| IBIS file stm32u535_545_ufqfpn48.ibs
[IBIS ver] 4.2
[File name] stm32u535_545_ufqfpn48.ibs
[File Rev] rev1.0
[Date]  11-09-2023
[Source] Data Created at STMicroelectronics
[Notes]  File originated from ELDO simulations.
[Disclaimer]  This information is for modeling purpose only and is
   not guaranteed. The information is subject to change without
   notice.
[Copyright] Copyright 2023 STMicroelectronics Inc.
|   Component stm32u535_545_ufqfpn48
[Component] stm32u535_545_ufqfpn48
[Manufacturer] STMicroelectronics
[Package]
| variable   typ   min   max
R_pkg  0  NA  NA
L_pkg  0  NA  NA
C_pkg  0  NA  NA
[Pin]   signal_name   model_name
1  VBAT  power
2  PC13  io8_100m_ft_v33
3  PC14-OSC32_IN  io8_100m_tamp_ft
4  PC15-OSC32_OUT  io8_100m_tamp_ft
5  PH0-OSC_IN  io8_100m_ft
6  PH1-OSC_OUT  io8_100m_ft
7  NRST  nc
8  VSSA  nc
9  VDDA  power
10  PA0  io8_100m_hslv_tamp_ft
11  PA1  io8_100m_hslv_tamp_ft
12  PA2  io8_100m_hslv_ft
13  PA3  io8_166m_hslv_ft
14  PA4  io8_100m_hslv_ft
15  PA5  io8_100m_ft
16  PA6  io8_100m_hslv_ft
17  PA7  io8_100m_hslv_i2c_ft
18  PB0  io8_100m_hslv_ft
19  PB1  io8_100m_hslv_ft
20  PB2  io8_100m_hslv_tamp_ft
21  PB10  io8_166m_hslv_i2c_ft
22  VCAP  nc
23  VSS  gnd
24  VDD  power
25  PB12  io8_166m_hslv_ft
26  PB13  io8_100m_i2c_ft
27  PB14  io8_100m_i2c_ft
28  PB15  io8_100m_ft
29  PA8  io8_166m_hslv_ft
30  PA9  io8_100m_ft
31  PA10  io8_100m_ft
32  PA11  io8_usb_ft
33  PA12  io8_usb_ft
34  PA13  io8_100m_ft
35  VSS  gnd
36  VDD  power
37  PA14  io8_100m_ft
38  PA15  io8_100m_ft
39  PB3  io8_100m_i2c_ft
40  PB4  io8_100m_i2c_ft
41  PB5  io8_166m_hslv_ft
42  PB6  io8_100m_i2c_ft
43  PB7  io8_166m_hslv_i2c_ft
44  PH3-BOOT0  io8_100m_ft
45  PB8  io8_100m_hslv_i2c_ft
46  PB9  io8_100m_hslv_i2c_ft
47  VSS  gnd
48  VDD  power
[Package Model]   455-qfpn-7x7-48-ldo-230504
[Pin Mapping]   pulldown_ref   pullup_ref   | Comment
1  nc  vsw
2  gndio  vddiom  | Depending on IO usage
| 2  gndio  vsw  | Depending on IO usage
3  gndio  vddiom  | Depending on IO usage
| 3  gndio  vsw  | Depending on IO usage
4  gndio  vddiom  | Depending on IO usage
| 4  gndio  vsw  | Depending on IO usage
5  gndio  vddiom
6  gndio  vddiom
7  nc   nc
8  nc  nc
9  nc  vddiom
10  gndio  vddiom
11  gndio  vddiom
12  gndio  vddiom
13  gndio  vddiom
14  gndio  vddiom
15  gndio  vddiom
16  gndio  vddiom
17  gndio  vddiom
18  gndio  vddiom
19  gndio  vddiom
20  gndio  vddiom
21  gndio  vddiom
22  nc  nc
23  gndio  nc
24  nc  vddiom
25  gndio  vddiom
26  gndio  vddiom
27  gndio  vddiom
28  gndio  vddiom
29  gndio  vddiom
30  gndio  vddiom  | Depending on IO usage
| 30  gndio  vddusb  | Depending on IO usage
31  gndio  vddiom  | Depending on IO usage
| 31  gndio  vddusb  | Depending on IO usage
32  gndio  vddiom  | Depending on IO usage
| 32  gndio  vddusb  | Depending on IO usage
33  gndio  vddiom  | Depending on IO usage
| 33  gndio  vddusb  | Depending on IO usage
34  gndio  vddiom  | Depending on IO usage
| 34  gndio  vddusb  | Depending on IO usage
35  gndio  nc
36  nc  vddiom
37  gndio  vddiom
38  gndio  vddiom
39  gndio  vddiom
40  gndio  vddiom
41  gndio  vddiom
42  gndio  vddiom
43  gndio  vddiom
44  gndio  vddiom
45  gndio  vddiom
46  gndio  vddiom
47  gndio  nc
48  nc  vddiom
[Model Selector] io8_100m_ft
io8_100m_ft_hs_1v2  "IO8_FT 100MHz high speed @ 1.2V"
io8_100m_ft_fs_1v2  "IO8_FT 100MHz fast speed @ 1.2V"
io8_100m_ft_fs_pd_1v2  "IO8_FT 100MHz fast speed @ 1.2V pulldown"
io8_100m_ft_ms_1v2  "IO8_FT 100MHz med speed @ 1.2V"
io8_100m_ft_ms_pd_1v2  "IO8_FT 100MHz med speed @ 1.2V pulldown"
io8_100m_ft_ls_1v2  "IO8_FT 100MHz low speed @ 1.2V"
io8_100m_ft_ls_pd_1v2  "IO8_FT 100MHz low speed @ 1.2V pulldown"
io8_100m_ft_hs_1v8  "IO8_FT 100MHz high speed @ 1.8V"
io8_100m_ft_hs_pd_1v8  "IO8_FT 100MHz high speed @ 1.8V pulldown"
io8_100m_ft_fs_1v8  "IO8_FT 100MHz fast speed @ 1.8V"
io8_100m_ft_fs_pd_1v8  "IO8_FT 100MHz fast speed @ 1.8V pulldown"
io8_100m_ft_ms_1v8  "IO8_FT 100MHz med speed @ 1.8V"
io8_100m_ft_ms_pd_1v8  "IO8_FT 100MHz med speed @ 1.8V pulldown"
io8_100m_ft_ls_1v8  "IO8_FT 100MHz low speed @ 1.8V"
io8_100m_ft_ls_pd_1v8  "IO8_FT 100MHz low speed @ 1.8V pulldown"
io8_100m_ft_hs_3v3  "IO8_FT 100MHz high speed @ 3.3V"
io8_100m_ft_hs_pd_3v3  "IO8_FT 100MHz high speed @ 3.3V pulldown"
io8_100m_ft_fs_3v3  "IO8_FT 100MHz fast speed @ 3.3V"
io8_100m_ft_fs_pd_3v3  "IO8_FT 100MHz fast speed @ 3.3V pulldown"
io8_100m_ft_ms_3v3  "IO8_FT 100MHz med speed @ 3.3V"
io8_100m_ft_ms_pd_3v3  "IO8_FT 100MHz med speed @ 3.3V pulldown"
io8_100m_ft_ls_3v3  "IO8_FT 100MHz low speed @ 3.3V"
io8_100m_ft_ls_pd_3v3  "IO8_FT 100MHz low speed @ 3.3V pulldown"
[Model Selector] io8_100m_hslv_ft
io8_100m_ft_hs_1v2  "IO8_FT 100MHz high speed @ 1.2V"
io8_100m_ft_hs_pu_1v2  "IO8_FT 100MHz high speed @ 1.2V pullup"
io8_100m_ft_hs_pd_1v2  "IO8_FT 100MHz high speed @ 1.2V pulldown"
io8_100m_ft_fs_1v2  "IO8_FT 100MHz fast speed @ 1.2V"
io8_100m_ft_fs_pu_1v2  "IO8_FT 100MHz fast speed @ 1.2V pullup"
io8_100m_ft_fs_pd_1v2  "IO8_FT 100MHz fast speed @ 1.2V pulldown"
io8_100m_ft_ms_1v2  "IO8_FT 100MHz med speed @ 1.2V"
io8_100m_ft_ms_pu_1v2  "IO8_FT 100MHz med speed @ 1.2V pullup"
io8_100m_ft_ms_pd_1v2  "IO8_FT 100MHz med speed @ 1.2V pulldown"
io8_100m_ft_ls_1v2  "IO8_FT 100MHz low speed @ 1.2V"
io8_100m_ft_ls_pu_1v2  "IO8_FT 100MHz low speed @ 1.2V pullup"
io8_100m_ft_ls_pd_1v2  "IO8_FT 100MHz low speed @ 1.2V pulldown"
io8_100m_ft_hs_1v8  "IO8_FT 100MHz high speed @ 1.8V"
io8_100m_ft_hs_pu_1v8  "IO8_FT 100MHz high speed @ 1.8V pullup"
io8_100m_ft_hs_pd_1v8  "IO8_FT 100MHz high speed @ 1.8V pulldown"
io8_100m_ft_fs_1v8  "IO8_FT 100MHz fast speed @ 1.8V"
io8_100m_ft_fs_pu_1v8  "IO8_FT 100MHz fast speed @ 1.8V pullup"
io8_100m_ft_fs_pd_1v8  "IO8_FT 100MHz fast speed @ 1.8V pulldown"
io8_100m_ft_ms_1v8  "IO8_FT 100MHz med speed @ 1.8V"
io8_100m_ft_ms_pu_1v8  "IO8_FT 100MHz med speed @ 1.8V pullup"
io8_100m_ft_ms_pd_1v8  "IO8_FT 100MHz med speed @ 1.8V pulldown"
io8_100m_ft_ls_1v8  "IO8_FT 100MHz low speed @ 1.8V"
io8_100m_ft_ls_pu_1v8  "IO8_FT 100MHz low speed @ 1.8V pullup"
io8_100m_ft_ls_pd_1v8  "IO8_FT 100MHz low speed @ 1.8V pulldown"
io8_100m_ft_hs_3v3  "IO8_FT 100MHz high speed @ 3.3V"
io8_100m_ft_hs_pu_3v3  "IO8_FT 100MHz high speed @ 3.3V pullup"
io8_100m_ft_hs_pd_3v3  "IO8_FT 100MHz high speed @ 3.3V pulldown"
io8_100m_ft_fs_3v3  "IO8_FT 100MHz fast speed @ 3.3V"
io8_100m_ft_fs_pu_3v3  "IO8_FT 100MHz fast speed @ 3.3V pullup"
io8_100m_ft_fs_pd_3v3  "IO8_FT 100MHz fast speed @ 3.3V pulldown"
io8_100m_ft_ms_3v3  "IO8_FT 100MHz med speed @ 3.3V"
io8_100m_ft_ms_pu_3v3  "IO8_FT 100MHz med speed @ 3.3V pullup"
io8_100m_ft_ms_pd_3v3  "IO8_FT 100MHz med speed @ 3.3V pulldown"
io8_100m_ft_ls_3v3  "IO8_FT 100MHz low speed @ 3.3V"
io8_100m_ft_ls_pu_3v3  "IO8_FT 100MHz low speed @ 3.3V pullup"
io8_100m_ft_ls_pd_3v3  "IO8_FT 100MHz low speed @ 3.3V pulldown"
io8_100m_hslv_ft_hs_1v2  "IO8_FT 100MHz HSLV high speed @ 1.2V"
io8_100m_hslv_ft_hs_pu_1v2  "IO8_FT 100MHz HSLV high speed @ 1.2V pullup"
io8_100m_hslv_ft_hs_pd_1v2  "IO8_FT 100MHz HSLV high speed @ 1.2V pulldown"
io8_100m_hslv_ft_fs_1v2  "IO8_FT 100MHz HSLV fast speed @ 1.2V"
io8_100m_hslv_ft_fs_pu_1v2  "IO8_FT 100MHz HSLV fast speed @ 1.2V pullup"
io8_100m_hslv_ft_fs_pd_1v2  "IO8_FT 100MHz HSLV fast speed @ 1.2V pulldown"
io8_100m_hslv_ft_ms_1v2  "IO8_FT 100MHz HSLV med speed @ 1.2V"
io8_100m_hslv_ft_ms_pu_1v2  "IO8_FT 100MHz HSLV med speed @ 1.2V pullup"
io8_100m_hslv_ft_ms_pd_1v2  "IO8_FT 100MHz HSLV med speed @ 1.2V pulldown"
io8_100m_hslv_ft_ls_1v2  "IO8_FT 100MHz HSLV low speed @ 1.2V"
io8_100m_hslv_ft_ls_pu_1v2  "IO8_FT 100MHz HSLV low speed @ 1.2V pullup"
io8_100m_hslv_ft_ls_pd_1v2  "IO8_FT 100MHz HSLV low speed @ 1.2V pulldown"
io8_100m_hslv_ft_hs_1v8  "IO8_FT 100MHz HSLV high speed @ 1.8V"
io8_100m_hslv_ft_hs_pu_1v8  "IO8_FT 100MHz HSLV high speed @ 1.8V pullup"
io8_100m_hslv_ft_hs_pd_1v8  "IO8_FT 100MHz HSLV high speed @ 1.8V pulldown"
io8_100m_hslv_ft_fs_1v8  "IO8_FT 100MHz HSLV fast speed @ 1.8V"
io8_100m_hslv_ft_fs_pu_1v8  "IO8_FT 100MHz HSLV fast speed @ 1.8V pullup"
io8_100m_hslv_ft_fs_pd_1v8  "IO8_FT 100MHz HSLV fast speed @ 1.8V pulldown"
io8_100m_hslv_ft_ms_1v8  "IO8_FT 100MHz HSLV med speed @ 1.8V"
io8_100m_hslv_ft_ms_pu_1v8  "IO8_FT 100MHz HSLV med speed @ 1.8V pullup"
io8_100m_hslv_ft_ms_pd_1v8  "IO8_FT 100MHz HSLV med speed @ 1.8V pulldown"
io8_100m_hslv_ft_ls_1v8  "IO8_FT 100MHz HSLV low speed @ 1.8V"
io8_100m_hslv_ft_ls_pu_1v8  "IO8_FT 100MHz HSLV low speed @ 1.8V pullup"
io8_100m_hslv_ft_ls_pd_1v8  "IO8_FT 100MHz HSLV low speed @ 1.8V pulldown"
io8_100m_hslv_ft_hs_2v5  "IO8_FT 100MHz HSLV high speed @ 2.5V"
io8_100m_hslv_ft_hs_pu_2v5  "IO8_FT 100MHz HSLV high speed @ 2.5V pullup"
io8_100m_hslv_ft_hs_pd_2v5  "IO8_FT 100MHz HSLV high speed @ 2.5V pulldown"
io8_100m_hslv_ft_fs_2v5  "IO8_FT 100MHz HSLV fast speed @ 2.5V"
io8_100m_hslv_ft_fs_pu_2v5  "IO8_FT 100MHz HSLV fast speed @ 2.5V pullup"
io8_100m_hslv_ft_fs_pd_2v5  "IO8_FT 100MHz HSLV fast speed @ 2.5V pulldown"
io8_100m_hslv_ft_ms_2v5  "IO8_FT 100MHz HSLV med speed @ 2.5V"
io8_100m_hslv_ft_ms_pu_2v5  "IO8_FT 100MHz HSLV med speed @ 2.5V pullup"
io8_100m_hslv_ft_ms_pd_2v5  "IO8_FT 100MHz HSLV med speed @ 2.5V pulldown"
io8_100m_hslv_ft_ls_2v5  "IO8_FT 100MHz HSLV low speed @ 2.5V"
io8_100m_hslv_ft_ls_pu_2v5  "IO8_FT 100MHz HSLV low speed @ 2.5V pullup"
io8_100m_hslv_ft_ls_pd_2v5  "IO8_FT 100MHz HSLV low speed @ 2.5V pulldown"
[Model Selector] io8_100m_hslv_i2c_ft
io8_100m_ft_hs_1v2  "IO8_FT 100MHz high speed @ 1.2V"
io8_100m_ft_hs_pu_1v2  "IO8_FT 100MHz high speed @ 1.2V pullup"
io8_100m_ft_hs_pd_1v2  "IO8_FT 100MHz high speed @ 1.2V pulldown"
io8_100m_ft_fs_1v2  "IO8_FT 100MHz fast speed @ 1.2V"
io8_100m_ft_fs_pu_1v2  "IO8_FT 100MHz fast speed @ 1.2V pullup"
io8_100m_ft_fs_pd_1v2  "IO8_FT 100MHz fast speed @ 1.2V pulldown"
io8_100m_ft_ms_1v2  "IO8_FT 100MHz med speed @ 1.2V"
io8_100m_ft_ms_pu_1v2  "IO8_FT 100MHz med speed @ 1.2V pullup"
io8_100m_ft_ms_pd_1v2  "IO8_FT 100MHz med speed @ 1.2V pulldown"
io8_100m_ft_ls_1v2  "IO8_FT 100MHz low speed @ 1.2V"
io8_100m_ft_ls_pu_1v2  "IO8_FT 100MHz low speed @ 1.2V pullup"
io8_100m_ft_ls_pd_1v2  "IO8_FT 100MHz low speed @ 1.2V pulldown"
io8_100m_ft_hs_1v8  "IO8_FT 100MHz high speed @ 1.8V"
io8_100m_ft_hs_pu_1v8  "IO8_FT 100MHz high speed @ 1.8V pullup"
io8_100m_ft_hs_pd_1v8  "IO8_FT 100MHz high speed @ 1.8V pulldown"
io8_100m_ft_fs_1v8  "IO8_FT 100MHz fast speed @ 1.8V"
io8_100m_ft_fs_pu_1v8  "IO8_FT 100MHz fast speed @ 1.8V pullup"
io8_100m_ft_fs_pd_1v8  "IO8_FT 100MHz fast speed @ 1.8V pulldown"
io8_100m_ft_ms_1v8  "IO8_FT 100MHz med speed @ 1.8V"
io8_100m_ft_ms_pu_1v8  "IO8_FT 100MHz med speed @ 1.8V pullup"
io8_100m_ft_ms_pd_1v8  "IO8_FT 100MHz med speed @ 1.8V pulldown"
io8_100m_ft_ls_1v8  "IO8_FT 100MHz low speed @ 1.8V"
io8_100m_ft_ls_pu_1v8  "IO8_FT 100MHz low speed @ 1.8V pullup"
io8_100m_ft_ls_pd_1v8  "IO8_FT 100MHz low speed @ 1.8V pulldown"
io8_100m_ft_hs_3v3  "IO8_FT 100MHz high speed @ 3.3V"
io8_100m_ft_hs_pu_3v3  "IO8_FT 100MHz high speed @ 3.3V pullup"
io8_100m_ft_hs_pd_3v3  "IO8_FT 100MHz high speed @ 3.3V pulldown"
io8_100m_ft_fs_3v3  "IO8_FT 100MHz fast speed @ 3.3V"
io8_100m_ft_fs_pu_3v3  "IO8_FT 100MHz fast speed @ 3.3V pullup"
io8_100m_ft_fs_pd_3v3  "IO8_FT 100MHz fast speed @ 3.3V pulldown"
io8_100m_ft_ms_3v3  "IO8_FT 100MHz med speed @ 3.3V"
io8_100m_ft_ms_pu_3v3  "IO8_FT 100MHz med speed @ 3.3V pullup"
io8_100m_ft_ms_pd_3v3  "IO8_FT 100MHz med speed @ 3.3V pulldown"
io8_100m_ft_ls_3v3  "IO8_FT 100MHz low speed @ 3.3V"
io8_100m_ft_ls_pu_3v3  "IO8_FT 100MHz low speed @ 3.3V pullup"
io8_100m_ft_ls_pd_3v3  "IO8_FT 100MHz low speed @ 3.3V pulldown"
io8_100m_hslv_ft_hs_1v2  "IO8_FT 100MHz HSLV high speed @ 1.2V"
io8_100m_hslv_ft_hs_pu_1v2  "IO8_FT 100MHz HSLV high speed @ 1.2V pullup"
io8_100m_hslv_ft_hs_pd_1v2  "IO8_FT 100MHz HSLV high speed @ 1.2V pulldown"
io8_100m_hslv_ft_fs_1v2  "IO8_FT 100MHz HSLV fast speed @ 1.2V"
io8_100m_hslv_ft_fs_pu_1v2  "IO8_FT 100MHz HSLV fast speed @ 1.2V pullup"
io8_100m_hslv_ft_fs_pd_1v2  "IO8_FT 100MHz HSLV fast speed @ 1.2V pulldown"
io8_100m_hslv_ft_ms_1v2  "IO8_FT 100MHz HSLV med speed @ 1.2V"
io8_100m_hslv_ft_ms_pu_1v2  "IO8_FT 100MHz HSLV med speed @ 1.2V pullup"
io8_100m_hslv_ft_ms_pd_1v2  "IO8_FT 100MHz HSLV med speed @ 1.2V pulldown"
io8_100m_hslv_ft_ls_1v2  "IO8_FT 100MHz HSLV low speed @ 1.2V"
io8_100m_hslv_ft_ls_pu_1v2  "IO8_FT 100MHz HSLV low speed @ 1.2V pullup"
io8_100m_hslv_ft_ls_pd_1v2  "IO8_FT 100MHz HSLV low speed @ 1.2V pulldown"
io8_100m_hslv_ft_hs_1v8  "IO8_FT 100MHz HSLV high speed @ 1.8V"
io8_100m_hslv_ft_hs_pu_1v8  "IO8_FT 100MHz HSLV high speed @ 1.8V pullup"
io8_100m_hslv_ft_hs_pd_1v8  "IO8_FT 100MHz HSLV high speed @ 1.8V pulldown"
io8_100m_hslv_ft_fs_1v8  "IO8_FT 100MHz HSLV fast speed @ 1.8V"
io8_100m_hslv_ft_fs_pu_1v8  "IO8_FT 100MHz HSLV fast speed @ 1.8V pullup"
io8_100m_hslv_ft_fs_pd_1v8  "IO8_FT 100MHz HSLV fast speed @ 1.8V pulldown"
io8_100m_hslv_ft_ms_1v8  "IO8_FT 100MHz HSLV med speed @ 1.8V"
io8_100m_hslv_ft_ms_pu_1v8  "IO8_FT 100MHz HSLV med speed @ 1.8V pullup"
io8_100m_hslv_ft_ms_pd_1v8  "IO8_FT 100MHz HSLV med speed @ 1.8V pulldown"
io8_100m_hslv_ft_ls_1v8  "IO8_FT 100MHz HSLV low speed @ 1.8V"
io8_100m_hslv_ft_ls_pu_1v8  "IO8_FT 100MHz HSLV low speed @ 1.8V pullup"
io8_100m_hslv_ft_ls_pd_1v8  "IO8_FT 100MHz HSLV low speed @ 1.8V pulldown"
io8_100m_hslv_ft_hs_2v5  "IO8_FT 100MHz HSLV high speed @ 2.5V"
io8_100m_hslv_ft_hs_pu_2v5  "IO8_FT 100MHz HSLV high speed @ 2.5V pullup"
io8_100m_hslv_ft_hs_pd_2v5  "IO8_FT 100MHz HSLV high speed @ 2.5V pulldown"
io8_100m_hslv_ft_fs_2v5  "IO8_FT 100MHz HSLV fast speed @ 2.5V"
io8_100m_hslv_ft_fs_pu_2v5  "IO8_FT 100MHz HSLV fast speed @ 2.5V pullup"
io8_100m_hslv_ft_fs_pd_2v5  "IO8_FT 100MHz HSLV fast speed @ 2.5V pulldown"
io8_100m_hslv_ft_ms_2v5  "IO8_FT 100MHz HSLV med speed @ 2.5V"
io8_100m_hslv_ft_ms_pu_2v5  "IO8_FT 100MHz HSLV med speed @ 2.5V pullup"
io8_100m_hslv_ft_ms_pd_2v5  "IO8_FT 100MHz HSLV med speed @ 2.5V pulldown"
io8_100m_hslv_ft_ls_2v5  "IO8_FT 100MHz HSLV low speed @ 2.5V"
io8_100m_hslv_ft_ls_pu_2v5  "IO8_FT 100MHz HSLV low speed @ 2.5V pullup"
io8_100m_hslv_ft_ls_pd_2v5  "IO8_FT 100MHz HSLV low speed @ 2.5V pulldown"
[Model Selector] io8_100m_hslv_tamp_ft
io8_100m_ft_hs_1v2  "IO8_FT 100MHz high speed @ 1.2V"
io8_100m_ft_hs_pu_1v2  "IO8_FT 100MHz high speed @ 1.2V pullup"
io8_100m_ft_hs_pd_1v2  "IO8_FT 100MHz high speed @ 1.2V pulldown"
io8_100m_ft_fs_1v2  "IO8_FT 100MHz fast speed @ 1.2V"
io8_100m_ft_fs_pu_1v2  "IO8_FT 100MHz fast speed @ 1.2V pullup"
io8_100m_ft_fs_pd_1v2  "IO8_FT 100MHz fast speed @ 1.2V pulldown"
io8_100m_ft_ms_1v2  "IO8_FT 100MHz med speed @ 1.2V"
io8_100m_ft_ms_pu_1v2  "IO8_FT 100MHz med speed @ 1.2V pullup"
io8_100m_ft_ms_pd_1v2  "IO8_FT 100MHz med speed @ 1.2V pulldown"
io8_100m_ft_ls_1v2  "IO8_FT 100MHz low speed @ 1.2V"
io8_100m_ft_ls_pu_1v2  "IO8_FT 100MHz low speed @ 1.2V pullup"
io8_100m_ft_ls_pd_1v2  "IO8_FT 100MHz low speed @ 1.2V pulldown"
io8_100m_ft_hs_1v8  "IO8_FT 100MHz high speed @ 1.8V"
io8_100m_ft_hs_pu_1v8  "IO8_FT 100MHz high speed @ 1.8V pullup"
io8_100m_ft_hs_pd_1v8  "IO8_FT 100MHz high speed @ 1.8V pulldown"
io8_100m_ft_fs_1v8  "IO8_FT 100MHz fast speed @ 1.8V"
io8_100m_ft_fs_pu_1v8  "IO8_FT 100MHz fast speed @ 1.8V pullup"
io8_100m_ft_fs_pd_1v8  "IO8_FT 100MHz fast speed @ 1.8V pulldown"
io8_100m_ft_ms_1v8  "IO8_FT 100MHz med speed @ 1.8V"
io8_100m_ft_ms_pu_1v8  "IO8_FT 100MHz med speed @ 1.8V pullup"
io8_100m_ft_ms_pd_1v8  "IO8_FT 100MHz med speed @ 1.8V pulldown"
io8_100m_ft_ls_1v8  "IO8_FT 100MHz low speed @ 1.8V"
io8_100m_ft_ls_pu_1v8  "IO8_FT 100MHz low speed @ 1.8V pullup"
io8_100m_ft_ls_pd_1v8  "IO8_FT 100MHz low speed @ 1.8V pulldown"
io8_100m_ft_hs_3v3  "IO8_FT 100MHz high speed @ 3.3V"
io8_100m_ft_hs_pu_3v3  "IO8_FT 100MHz high speed @ 3.3V pullup"
io8_100m_ft_hs_pd_3v3  "IO8_FT 100MHz high speed @ 3.3V pulldown"
io8_100m_ft_fs_3v3  "IO8_FT 100MHz fast speed @ 3.3V"
io8_100m_ft_fs_pu_3v3  "IO8_FT 100MHz fast speed @ 3.3V pullup"
io8_100m_ft_fs_pd_3v3  "IO8_FT 100MHz fast speed @ 3.3V pulldown"
io8_100m_ft_ms_3v3  "IO8_FT 100MHz med speed @ 3.3V"
io8_100m_ft_ms_pu_3v3  "IO8_FT 100MHz med speed @ 3.3V pullup"
io8_100m_ft_ms_pd_3v3  "IO8_FT 100MHz med speed @ 3.3V pulldown"
io8_100m_ft_ls_3v3  "IO8_FT 100MHz low speed @ 3.3V"
io8_100m_ft_ls_pu_3v3  "IO8_FT 100MHz low speed @ 3.3V pullup"
io8_100m_ft_ls_pd_3v3  "IO8_FT 100MHz low speed @ 3.3V pulldown"
io8_100m_hslv_ft_hs_1v2  "IO8_FT 100MHz HSLV high speed @ 1.2V"
io8_100m_hslv_ft_hs_pu_1v2  "IO8_FT 100MHz HSLV high speed @ 1.2V pullup"
io8_100m_hslv_ft_hs_pd_1v2  "IO8_FT 100MHz HSLV high speed @ 1.2V pulldown"
io8_100m_hslv_ft_fs_1v2  "IO8_FT 100MHz HSLV fast speed @ 1.2V"
io8_100m_hslv_ft_fs_pu_1v2  "IO8_FT 100MHz HSLV fast speed @ 1.2V pullup"
io8_100m_hslv_ft_fs_pd_1v2  "IO8_FT 100MHz HSLV fast speed @ 1.2V pulldown"
io8_100m_hslv_ft_ms_1v2  "IO8_FT 100MHz HSLV med speed @ 1.2V"
io8_100m_hslv_ft_ms_pu_1v2  "IO8_FT 100MHz HSLV med speed @ 1.2V pullup"
io8_100m_hslv_ft_ms_pd_1v2  "IO8_FT 100MHz HSLV med speed @ 1.2V pulldown"
io8_100m_hslv_ft_ls_1v2  "IO8_FT 100MHz HSLV low speed @ 1.2V"
io8_100m_hslv_ft_ls_pu_1v2  "IO8_FT 100MHz HSLV low speed @ 1.2V pullup"
io8_100m_hslv_ft_ls_pd_1v2  "IO8_FT 100MHz HSLV low speed @ 1.2V pulldown"
io8_100m_hslv_ft_hs_1v8  "IO8_FT 100MHz HSLV high speed @ 1.8V"
io8_100m_hslv_ft_hs_pu_1v8  "IO8_FT 100MHz HSLV high speed @ 1.8V pullup"
io8_100m_hslv_ft_hs_pd_1v8  "IO8_FT 100MHz HSLV high speed @ 1.8V pulldown"
io8_100m_hslv_ft_fs_1v8  "IO8_FT 100MHz HSLV fast speed @ 1.8V"
io8_100m_hslv_ft_fs_pu_1v8  "IO8_FT 100MHz HSLV fast speed @ 1.8V pullup"
io8_100m_hslv_ft_fs_pd_1v8  "IO8_FT 100MHz HSLV fast speed @ 1.8V pulldown"
io8_100m_hslv_ft_ms_1v8  "IO8_FT 100MHz HSLV med speed @ 1.8V"
io8_100m_hslv_ft_ms_pu_1v8  "IO8_FT 100MHz HSLV med speed @ 1.8V pullup"
io8_100m_hslv_ft_ms_pd_1v8  "IO8_FT 100MHz HSLV med speed @ 1.8V pulldown"
io8_100m_hslv_ft_ls_1v8  "IO8_FT 100MHz HSLV low speed @ 1.8V"
io8_100m_hslv_ft_ls_pu_1v8  "IO8_FT 100MHz HSLV low speed @ 1.8V pullup"
io8_100m_hslv_ft_ls_pd_1v8  "IO8_FT 100MHz HSLV low speed @ 1.8V pulldown"
io8_100m_hslv_ft_hs_2v5  "IO8_FT 100MHz HSLV high speed @ 2.5V"
io8_100m_hslv_ft_hs_pu_2v5  "IO8_FT 100MHz HSLV high speed @ 2.5V pullup"
io8_100m_hslv_ft_hs_pd_2v5  "IO8_FT 100MHz HSLV high speed @ 2.5V pulldown"
io8_100m_hslv_ft_fs_2v5  "IO8_FT 100MHz HSLV fast speed @ 2.5V"
io8_100m_hslv_ft_fs_pu_2v5  "IO8_FT 100MHz HSLV fast speed @ 2.5V pullup"
io8_100m_hslv_ft_fs_pd_2v5  "IO8_FT 100MHz HSLV fast speed @ 2.5V pulldown"
io8_100m_hslv_ft_ms_2v5  "IO8_FT 100MHz HSLV med speed @ 2.5V"
io8_100m_hslv_ft_ms_pu_2v5  "IO8_FT 100MHz HSLV med speed @ 2.5V pullup"
io8_100m_hslv_ft_ms_pd_2v5  "IO8_FT 100MHz HSLV med speed @ 2.5V pulldown"
io8_100m_hslv_ft_ls_2v5  "IO8_FT 100MHz HSLV low speed @ 2.5V"
io8_100m_hslv_ft_ls_pu_2v5  "IO8_FT 100MHz HSLV low speed @ 2.5V pullup"
io8_100m_hslv_ft_ls_pd_2v5  "IO8_FT 100MHz HSLV low speed @ 2.5V pulldown"
io8_ft_v33_hs_1v2  "IO8_FT_V33 high speed @ 1.2V"
io8_ft_v33_hs_pu_1v2  "IO8_FT_V33 high speed @ 1.2V pullup"
io8_ft_v33_hs_pd_1v2  "IO8_FT_V33 high speed @ 1.2V pulldown"
io8_ft_v33_fs_1v2  "IO8_FT_V33 fast speed @ 1.2V"
io8_ft_v33_fs_pu_1v2  "IO8_FT_V33 fast speed @ 1.2V pullup"
io8_ft_v33_fs_pd_1v2  "IO8_FT_V33 fast speed @ 1.2V pulldown"
io8_ft_v33_ms_1v2  "IO8_FT_V33 med speed @ 1.2V"
io8_ft_v33_ms_pu_1v2  "IO8_FT_V33 med speed @ 1.2V pullup"
io8_ft_v33_ms_pd_1v2  "IO8_FT_V33 med speed @ 1.2V pulldown"
io8_ft_v33_ls_1v2  "IO8_FT_V33 low speed @ 1.2V"
io8_ft_v33_ls_pu_1v2  "IO8_FT_V33 low speed @ 1.2V pullup"
io8_ft_v33_ls_pd_1v2  "IO8_FT_V33 low speed @ 1.2V pulldown"
io8_ft_v33_hs_1v8  "IO8_FT_V33 high speed @ 1.8V"
io8_ft_v33_hs_pu_1v8  "IO8_FT_V33 high speed @ 1.8V pullup"
io8_ft_v33_hs_pd_1v8  "IO8_FT_V33 high speed @ 1.8V pulldown"
io8_ft_v33_fs_1v8  "IO8_FT_V33 fast speed @ 1.8V"
io8_ft_v33_fs_pu_1v8  "IO8_FT_V33 fast speed @ 1.8V pullup"
io8_ft_v33_fs_pd_1v8  "IO8_FT_V33 fast speed @ 1.8V pulldown"
io8_ft_v33_ms_1v8  "IO8_FT_V33 med speed @ 1.8V"
io8_ft_v33_ms_pu_1v8  "IO8_FT_V33 med speed @ 1.8V pullup"
io8_ft_v33_ms_pd_1v8  "IO8_FT_V33 med speed @ 1.8V pulldown"
io8_ft_v33_ls_1v8  "IO8_FT_V33 low speed @ 1.8V"
io8_ft_v33_ls_pu_1v8  "IO8_FT_V33 low speed @ 1.8V pullup"
io8_ft_v33_ls_pd_1v8  "IO8_FT_V33 low speed @ 1.8V pulldown"
io8_ft_v33_hs_3v3  "IO8_FT_V33 high speed @ 3.3V"
io8_ft_v33_hs_pu_3v3  "IO8_FT_V33 high speed @ 3.3V pullup"
io8_ft_v33_hs_pd_3v3  "IO8_FT_V33 high speed @ 3.3V pulldown"
io8_ft_v33_fs_3v3  "IO8_FT_V33 fast speed @ 3.3V"
io8_ft_v33_fs_pu_3v3  "IO8_FT_V33 fast speed @ 3.3V pullup"
io8_ft_v33_fs_pd_3v3  "IO8_FT_V33 fast speed @ 3.3V pulldown"
io8_ft_v33_ms_3v3  "IO8_FT_V33 med speed @ 3.3V"
io8_ft_v33_ms_pu_3v3  "IO8_FT_V33 med speed @ 3.3V pullup"
io8_ft_v33_ms_pd_3v3  "IO8_FT_V33 med speed @ 3.3V pulldown"
io8_ft_v33_ls_3v3  "IO8_FT_V33 low speed @ 3.3V"
io8_ft_v33_ls_pu_3v3  "IO8_FT_V33 low speed @ 3.3V pullup"
io8_ft_v33_ls_pd_3v3  "IO8_FT_V33 low speed @ 3.3V pulldown"
[Model Selector] io8_100m_i2c_ft
io8_100m_ft_hs_1v2  "IO8_FT 100MHz high speed @ 1.2V"
io8_100m_ft_hs_pu_1v2  "IO8_FT 100MHz high speed @ 1.2V pullup"
io8_100m_ft_hs_pd_1v2  "IO8_FT 100MHz high speed @ 1.2V pulldown"
io8_100m_ft_fs_1v2  "IO8_FT 100MHz fast speed @ 1.2V"
io8_100m_ft_fs_pu_1v2  "IO8_FT 100MHz fast speed @ 1.2V pullup"
io8_100m_ft_fs_pd_1v2  "IO8_FT 100MHz fast speed @ 1.2V pulldown"
io8_100m_ft_ms_1v2  "IO8_FT 100MHz med speed @ 1.2V"
io8_100m_ft_ms_pu_1v2  "IO8_FT 100MHz med speed @ 1.2V pullup"
io8_100m_ft_ms_pd_1v2  "IO8_FT 100MHz med speed @ 1.2V pulldown"
io8_100m_ft_ls_1v2  "IO8_FT 100MHz low speed @ 1.2V"
io8_100m_ft_ls_pu_1v2  "IO8_FT 100MHz low speed @ 1.2V pullup"
io8_100m_ft_ls_pd_1v2  "IO8_FT 100MHz low speed @ 1.2V pulldown"
io8_100m_ft_hs_1v8  "IO8_FT 100MHz high speed @ 1.8V"
io8_100m_ft_hs_pu_1v8  "IO8_FT 100MHz high speed @ 1.8V pullup"
io8_100m_ft_hs_pd_1v8  "IO8_FT 100MHz high speed @ 1.8V pulldown"
io8_100m_ft_fs_1v8  "IO8_FT 100MHz fast speed @ 1.8V"
io8_100m_ft_fs_pu_1v8  "IO8_FT 100MHz fast speed @ 1.8V pullup"
io8_100m_ft_fs_pd_1v8  "IO8_FT 100MHz fast speed @ 1.8V pulldown"
io8_100m_ft_ms_1v8  "IO8_FT 100MHz med speed @ 1.8V"
io8_100m_ft_ms_pu_1v8  "IO8_FT 100MHz med speed @ 1.8V pullup"
io8_100m_ft_ms_pd_1v8  "IO8_FT 100MHz med speed @ 1.8V pulldown"
io8_100m_ft_ls_1v8  "IO8_FT 100MHz low speed @ 1.8V"
io8_100m_ft_ls_pu_1v8  "IO8_FT 100MHz low speed @ 1.8V pullup"
io8_100m_ft_ls_pd_1v8  "IO8_FT 100MHz low speed @ 1.8V pulldown"
io8_100m_ft_hs_3v3  "IO8_FT 100MHz high speed @ 3.3V"
io8_100m_ft_hs_pu_3v3  "IO8_FT 100MHz high speed @ 3.3V pullup"
io8_100m_ft_hs_pd_3v3  "IO8_FT 100MHz high speed @ 3.3V pulldown"
io8_100m_ft_fs_3v3  "IO8_FT 100MHz fast speed @ 3.3V"
io8_100m_ft_fs_pu_3v3  "IO8_FT 100MHz fast speed @ 3.3V pullup"
io8_100m_ft_fs_pd_3v3  "IO8_FT 100MHz fast speed @ 3.3V pulldown"
io8_100m_ft_ms_3v3  "IO8_FT 100MHz med speed @ 3.3V"
io8_100m_ft_ms_pu_3v3  "IO8_FT 100MHz med speed @ 3.3V pullup"
io8_100m_ft_ms_pd_3v3  "IO8_FT 100MHz med speed @ 3.3V pulldown"
io8_100m_ft_ls_3v3  "IO8_FT 100MHz low speed @ 3.3V"
io8_100m_ft_ls_pu_3v3  "IO8_FT 100MHz low speed @ 3.3V pullup"
io8_100m_ft_ls_pd_3v3  "IO8_FT 100MHz low speed @ 3.3V pulldown"
io8_100m_i2c_ft_1v2  "IO8_FT 100MHz I2C @ 1.2V"
io8_100m_i2c_ft_pu_1v2  "IO8_FT 100MHz I2C @ 1.2V pullup"
io8_100m_i2c_ft_pd_1v2  "IO8_FT 100MHz I2C @ 1.2V pulldown"
io8_100m_i2c_ft_1v8  "IO8_FT 100MHz I2C @ 1.8V"
io8_100m_i2c_ft_pu_1v8  "IO8_FT 100MHz I2C @ 1.8V pullup"
io8_100m_i2c_ft_pd_1v8  "IO8_FT 100MHz I2C @ 1,8V pulldown"
io8_100m_i2c_ft_3v3  "IO8_FT 100MHz I2C @ 3.3V"
io8_100m_i2c_ft_pu_3v3  "IO8_FT 100MHz I2C HSLV @ 3.3V pullup"
io8_100m_i2c_ft_pd_3v3  "IO8_FT 100MHz I2C @ 3.3V pulldown"
[Model Selector] io8_100m_tamp_ft
io8_100m_ft_hs_1v2  "IO8_FT 100MHz high speed @ 1.2V"
io8_100m_ft_hs_pu_1v2  "IO8_FT 100MHz high speed @ 1.2V pullup"
io8_100m_ft_hs_pd_1v2  "IO8_FT 100MHz high speed @ 1.2V pulldown"
io8_100m_ft_fs_1v2  "IO8_FT 100MHz fast speed @ 1.2V"
io8_100m_ft_fs_pu_1v2  "IO8_FT 100MHz fast speed @ 1.2V pullup"
io8_100m_ft_fs_pd_1v2  "IO8_FT 100MHz fast speed @ 1.2V pulldown"
io8_100m_ft_ms_1v2  "IO8_FT 100MHz med speed @ 1.2V"
io8_100m_ft_ms_pu_1v2  "IO8_FT 100MHz med speed @ 1.2V pullup"
io8_100m_ft_ms_pd_1v2  "IO8_FT 100MHz med speed @ 1.2V pulldown"
io8_100m_ft_ls_1v2  "IO8_FT 100MHz low speed @ 1.2V"
io8_100m_ft_ls_pu_1v2  "IO8_FT 100MHz low speed @ 1.2V pullup"
io8_100m_ft_ls_pd_1v2  "IO8_FT 100MHz low speed @ 1.2V pulldown"
io8_100m_ft_hs_1v8  "IO8_FT 100MHz high speed @ 1.8V"
io8_100m_ft_hs_pu_1v8  "IO8_FT 100MHz high speed @ 1.8V pullup"
io8_100m_ft_hs_pd_1v8  "IO8_FT 100MHz high speed @ 1.8V pulldown"
io8_100m_ft_fs_1v8  "IO8_FT 100MHz fast speed @ 1.8V"
io8_100m_ft_fs_pu_1v8  "IO8_FT 100MHz fast speed @ 1.8V pullup"
io8_100m_ft_fs_pd_1v8  "IO8_FT 100MHz fast speed @ 1.8V pulldown"
io8_100m_ft_ms_1v8  "IO8_FT 100MHz med speed @ 1.8V"
io8_100m_ft_ms_pu_1v8  "IO8_FT 100MHz med speed @ 1.8V pullup"
io8_100m_ft_ms_pd_1v8  "IO8_FT 100MHz med speed @ 1.8V pulldown"
io8_100m_ft_ls_1v8  "IO8_FT 100MHz low speed @ 1.8V"
io8_100m_ft_ls_pu_1v8  "IO8_FT 100MHz low speed @ 1.8V pullup"
io8_100m_ft_ls_pd_1v8  "IO8_FT 100MHz low speed @ 1.8V pulldown"
io8_100m_ft_hs_3v3  "IO8_FT 100MHz high speed @ 3.3V"
io8_100m_ft_hs_pu_3v3  "IO8_FT 100MHz high speed @ 3.3V pullup"
io8_100m_ft_hs_pd_3v3  "IO8_FT 100MHz high speed @ 3.3V pulldown"
io8_100m_ft_fs_3v3  "IO8_FT 100MHz fast speed @ 3.3V"
io8_100m_ft_fs_pu_3v3  "IO8_FT 100MHz fast speed @ 3.3V pullup"
io8_100m_ft_fs_pd_3v3  "IO8_FT 100MHz fast speed @ 3.3V pulldown"
io8_100m_ft_ms_3v3  "IO8_FT 100MHz med speed @ 3.3V"
io8_100m_ft_ms_pu_3v3  "IO8_FT 100MHz med speed @ 3.3V pullup"
io8_100m_ft_ms_pd_3v3  "IO8_FT 100MHz med speed @ 3.3V pulldown"
io8_100m_ft_ls_3v3  "IO8_FT 100MHz low speed @ 3.3V"
io8_100m_ft_ls_pu_3v3  "IO8_FT 100MHz low speed @ 3.3V pullup"
io8_100m_ft_ls_pd_3v3  "IO8_FT 100MHz low speed @ 3.3V pulldown"
io8_ft_v33_hs_1v2  "IO8_FT_V33 high speed @ 1.2V"
io8_ft_v33_hs_pu_1v2  "IO8_FT_V33 high speed @ 1.2V pullup"
io8_ft_v33_hs_pd_1v2  "IO8_FT_V33 high speed @ 1.2V pulldown"
io8_ft_v33_fs_1v2  "IO8_FT_V33 fast speed @ 1.2V"
io8_ft_v33_fs_pu_1v2  "IO8_FT_V33 fast speed @ 1.2V pullup"
io8_ft_v33_fs_pd_1v2  "IO8_FT_V33 fast speed @ 1.2V pulldown"
io8_ft_v33_ms_1v2  "IO8_FT_V33 med speed @ 1.2V"
io8_ft_v33_ms_pu_1v2  "IO8_FT_V33 med speed @ 1.2V pullup"
io8_ft_v33_ms_pd_1v2  "IO8_FT_V33 med speed @ 1.2V pulldown"
io8_ft_v33_ls_1v2  "IO8_FT_V33 low speed @ 1.2V"
io8_ft_v33_ls_pu_1v2  "IO8_FT_V33 low speed @ 1.2V pullup"
io8_ft_v33_ls_pd_1v2  "IO8_FT_V33 low speed @ 1.2V pulldown"
io8_ft_v33_hs_1v8  "IO8_FT_V33 high speed @ 1.8V"
io8_ft_v33_hs_pu_1v8  "IO8_FT_V33 high speed @ 1.8V pullup"
io8_ft_v33_hs_pd_1v8  "IO8_FT_V33 high speed @ 1.8V pulldown"
io8_ft_v33_fs_1v8  "IO8_FT_V33 fast speed @ 1.8V"
io8_ft_v33_fs_pu_1v8  "IO8_FT_V33 fast speed @ 1.8V pullup"
io8_ft_v33_fs_pd_1v8  "IO8_FT_V33 fast speed @ 1.8V pulldown"
io8_ft_v33_ms_1v8  "IO8_FT_V33 med speed @ 1.8V"
io8_ft_v33_ms_pu_1v8  "IO8_FT_V33 med speed @ 1.8V pullup"
io8_ft_v33_ms_pd_1v8  "IO8_FT_V33 med speed @ 1.8V pulldown"
io8_ft_v33_ls_1v8  "IO8_FT_V33 low speed @ 1.8V"
io8_ft_v33_ls_pu_1v8  "IO8_FT_V33 low speed @ 1.8V pullup"
io8_ft_v33_ls_pd_1v8  "IO8_FT_V33 low speed @ 1.8V pulldown"
io8_ft_v33_hs_3v3  "IO8_FT_V33 high speed @ 3.3V"
io8_ft_v33_hs_pu_3v3  "IO8_FT_V33 high speed @ 3.3V pullup"
io8_ft_v33_hs_pd_3v3  "IO8_FT_V33 high speed @ 3.3V pulldown"
io8_ft_v33_fs_3v3  "IO8_FT_V33 fast speed @ 3.3V"
io8_ft_v33_fs_pu_3v3  "IO8_FT_V33 fast speed @ 3.3V pullup"
io8_ft_v33_fs_pd_3v3  "IO8_FT_V33 fast speed @ 3.3V pulldown"
io8_ft_v33_ms_3v3  "IO8_FT_V33 med speed @ 3.3V"
io8_ft_v33_ms_pu_3v3  "IO8_FT_V33 med speed @ 3.3V pullup"
io8_ft_v33_ms_pd_3v3  "IO8_FT_V33 med speed @ 3.3V pulldown"
io8_ft_v33_ls_3v3  "IO8_FT_V33 low speed @ 3.3V"
io8_ft_v33_ls_pu_3v3  "IO8_FT_V33 low speed @ 3.3V pullup"
io8_ft_v33_ls_pd_3v3  "IO8_FT_V33 low speed @ 3.3V pulldown"
[Model Selector] io8_usb_ft
io8_100m_ft_hs_1v2  "IO8_FT 100MHz high speed @ 1.2V"
io8_100m_ft_hs_pu_1v2  "IO8_FT 100MHz high speed @ 1.2V pullup"
io8_100m_ft_hs_pd_1v2  "IO8_FT 100MHz high speed @ 1.2V pulldown"
io8_100m_ft_fs_1v2  "IO8_FT 100MHz fast speed @ 1.2V"
io8_100m_ft_fs_pu_1v2  "IO8_FT 100MHz fast speed @ 1.2V pullup"
io8_100m_ft_fs_pd_1v2  "IO8_FT 100MHz fast speed @ 1.2V pulldown"
io8_100m_ft_ms_1v2  "IO8_FT 100MHz med speed @ 1.2V"
io8_100m_ft_ms_pu_1v2  "IO8_FT 100MHz med speed @ 1.2V pullup"
io8_100m_ft_ms_pd_1v2  "IO8_FT 100MHz med speed @ 1.2V pulldown"
io8_100m_ft_ls_1v2  "IO8_FT 100MHz low speed @ 1.2V"
io8_100m_ft_ls_pu_1v2  "IO8_FT 100MHz low speed @ 1.2V pullup"
io8_100m_ft_ls_pd_1v2  "IO8_FT 100MHz low speed @ 1.2V pulldown"
io8_100m_ft_hs_1v8  "IO8_FT 100MHz high speed @ 1.8V"
io8_100m_ft_hs_pu_1v8  "IO8_FT 100MHz high speed @ 1.8V pullup"
io8_100m_ft_hs_pd_1v8  "IO8_FT 100MHz high speed @ 1.8V pulldown"
io8_100m_ft_fs_1v8  "IO8_FT 100MHz fast speed @ 1.8V"
io8_100m_ft_fs_pu_1v8  "IO8_FT 100MHz fast speed @ 1.8V pullup"
io8_100m_ft_fs_pd_1v8  "IO8_FT 100MHz fast speed @ 1.8V pulldown"
io8_100m_ft_ms_1v8  "IO8_FT 100MHz med speed @ 1.8V"
io8_100m_ft_ms_pu_1v8  "IO8_FT 100MHz med speed @ 1.8V pullup"
io8_100m_ft_ms_pd_1v8  "IO8_FT 100MHz med speed @ 1.8V pulldown"
io8_100m_ft_ls_1v8  "IO8_FT 100MHz low speed @ 1.8V"
io8_100m_ft_ls_pu_1v8  "IO8_FT 100MHz low speed @ 1.8V pullup"
io8_100m_ft_ls_pd_1v8  "IO8_FT 100MHz low speed @ 1.8V pulldown"
io8_100m_ft_hs_3v3  "IO8_FT 100MHz high speed @ 3.3V"
io8_100m_ft_hs_pu_3v3  "IO8_FT 100MHz high speed @ 3.3V pullup"
io8_100m_ft_hs_pd_3v3  "IO8_FT 100MHz high speed @ 3.3V pulldown"
io8_100m_ft_fs_3v3  "IO8_FT 100MHz fast speed @ 3.3V"
io8_100m_ft_fs_pu_3v3  "IO8_FT 100MHz fast speed @ 3.3V pullup"
io8_100m_ft_fs_pd_3v3  "IO8_FT 100MHz fast speed @ 3.3V pulldown"
io8_100m_ft_ms_3v3  "IO8_FT 100MHz med speed @ 3.3V"
io8_100m_ft_ms_pu_3v3  "IO8_FT 100MHz med speed @ 3.3V pullup"
io8_100m_ft_ms_pd_3v3  "IO8_FT 100MHz med speed @ 3.3V pulldown"
io8_100m_ft_ls_3v3  "IO8_FT 100MHz low speed @ 3.3V"
io8_100m_ft_ls_pu_3v3  "IO8_FT 100MHz low speed @ 3.3V pullup"
io8_100m_ft_ls_pd_3v3  "IO8_FT 100MHz low speed @ 3.3V pulldown"
io8_usb_fs_3v3  "IOUSB fast speed @ 3.3V"
io8_usb_fs_pu1_3v3  "IO8USB fast speed @ 3.3V pullup1"
io8_usb_fs_pd1_3v3  "IOUSB fast speed @ 3.3V pulldown1"
io8_usb_ls_3v3  "IOUSB low speed @ 3.3V"
io8_usb_ls_pu1_3v3  "IOUSB low speed @ 3.3V pullup1"
io8_usb_ls_pd1_3v3  "IOUSB low speed @ 3.3V pulldown1"
io8_usb_fs_pu2_3v3  "IOUSB fast speed @ 3.3V pullup2"
io8_usb_fs_pd2_3v3  "IOUSB fast speed @ 3.3V pulldown2"
io8_usb_ls_pu2_3v3  "IOUSB low speed @ 3.3V pullup2"
io8_usb_ls_pd2_3v3  "IOUSB low speed @ 3.3V pulldown2"
[Model Selector] io8_166m_hslv_ft
io8_166m_ft_hs_1v2  "IO8_FT 166MHz high speed @ 1.2V"
io8_166m_ft_hs_pu_1v2  "IO8_FT 166MHz high speed @ 1.2V pullup"
io8_166m_ft_hs_pd_1v2  "IO8_FT 166MHz high speed @ 1.2V pulldown"
io8_166m_ft_fs_1v2  "IO8_FT 166MHz fast speed @ 1.2V"
io8_166m_ft_fs_pu_1v2  "IO8_FT 166MHz fast speed @ 1.2V pullup"
io8_166m_ft_fs_pd_1v2  "IO8_FT 166MHz fast speed @ 1.2V pulldown"
io8_166m_ft_ms_1v2  "IO8_FT 166MHz med speed @ 1.2V"
io8_166m_ft_ms_pu_1v2  "IO8_FT 166MHz med speed @ 1.2V pullup"
io8_166m_ft_ms_pd_1v2  "IO8_FT 166MHz med speed @ 1.2V pulldown"
io8_166m_ft_ls_1v2  "IO8_FT 166MHz low speed @ 1.2V"
io8_166m_ft_ls_pu_1v2  "IO8_FT 166MHz low speed @ 1.2V pullup"
io8_166m_ft_ls_pd_1v2  "IO8_FT 166MHz low speed @ 1.2V pulldown"
io8_166m_ft_hs_1v8  "IO8_FT 166MHz high speed @ 1.8V"
io8_166m_ft_hs_pu_1v8  "IO8_FT 166MHz high speed @ 1.8V pullup"
io8_166m_ft_hs_pd_1v8  "IO8_FT 166MHz high speed @ 1.8V pulldown"
io8_166m_ft_fs_1v8  "IO8_FT 166MHz fast speed @ 1.8V"
io8_166m_ft_fs_pu_1v8  "IO8_FT 166MHz fast speed @ 1.8V pullup"
io8_166m_ft_fs_pd_1v8  "IO8_FT 166MHz fast speed @ 1.8V pulldown"
io8_166m_ft_ms_1v8  "IO8_FT 166MHz med speed @ 1.8V"
io8_166m_ft_ms_pu_1v8  "IO8_FT 166MHz med speed @ 1.8V pullup"
io8_166m_ft_ms_pd_1v8  "IO8_FT 166MHz med speed @ 1.8V pulldown"
io8_166m_ft_ls_1v8  "IO8_FT 166MHz low speed @ 1.8V"
io8_166m_ft_ls_pu_1v8  "IO8_FT 166MHz low speed @ 1.8V pullup"
io8_166m_ft_ls_pd_1v8  "IO8_FT 166MHz low speed @ 1.8V pulldown"
io8_166m_ft_hs_3v3  "IO8_FT 166MHz high speed @ 3.3V"
io8_166m_ft_hs_pu_3v3  "IO8_FT 166MHz high speed @ 3.3V pullup"
io8_166m_ft_hs_pd_3v3  "IO8_FT 166MHz high speed @ 3.3V pulldown"
io8_166m_ft_fs_3v3  "IO8_FT 166MHz fast speed @ 3.3V"
io8_166m_ft_fs_pu_3v3  "IO8_FT 166MHz fast speed @ 3.3V pullup"
io8_166m_ft_fs_pd_3v3  "IO8_FT 166MHz fast speed @ 3.3V pulldown"
io8_166m_ft_ms_3v3  "IO8_FT 166MHz med speed @ 3.3V"
io8_166m_ft_ms_pu_3v3  "IO8_FT 166MHz med speed @ 3.3V pullup"
io8_166m_ft_ms_pd_3v3  "IO8_FT 166MHz med speed @ 3.3V pulldown"
io8_166m_ft_ls_3v3  "IO8_FT 166MHz low speed @ 3.3V"
io8_166m_ft_ls_pu_3v3  "IO8_FT 166MHz low speed @ 3.3V pullup"
io8_166m_ft_ls_pd_3v3  "IO8_FT 166MHz low speed @ 3.3V pulldown"
io8_166m_hslv_ft_hs_1v2  "IO8_FT 166MHz HSLV high speed @ 1.2V"
io8_166m_hslv_ft_hs_pu_1v2  "IO8_FT 166MHz HSLV high speed @ 1.2V pullup"
io8_166m_hslv_ft_hs_pd_1v2  "IO8_FT 166MHz HSLV high speed @ 1.2V pulldown"
io8_166m_hslv_ft_fs_1v2  "IO8_FT 166MHz HSLV fast speed @ 1.2V"
io8_166m_hslv_ft_fs_pu_1v2  "IO8_FT 166MHz HSLV fast speed @ 1.2V pullup"
io8_166m_hslv_ft_fs_pd_1v2  "IO8_FT 166MHz HSLV fast speed @ 1.2V pulldown"
io8_166m_hslv_ft_ms_1v2  "IO8_FT 166MHz HSLV med speed @ 1.2V"
io8_166m_hslv_ft_ms_pu_1v2  "IO8_FT 166MHz HSLV med speed @ 1.2V pullup"
io8_166m_hslv_ft_ms_pd_1v2  "IO8_FT 166MHz HSLV med speed @ 1.2V pulldown"
io8_166m_hslv_ft_ls_1v2  "IO8_FT 166MHz HSLV low speed @ 1.2V"
io8_166m_hslv_ft_ls_pu_1v2  "IO8_FT 166MHz HSLV low speed @ 1.2V pullup"
io8_166m_hslv_ft_ls_pd_1v2  "IO8_FT 166MHz HSLV low speed @ 1.2V pulldown"
io8_166m_hslv_ft_hs_1v8  "IO8_FT 166MHz HSLV high speed @ 1.8V"
io8_166m_hslv_ft_hs_pu_1v8  "IO8_FT 166MHz HSLV high speed @ 1.8V pullup"
io8_166m_hslv_ft_hs_pd_1v8  "IO8_FT 166MHz HSLV high speed @ 1.8V pulldown"
io8_166m_hslv_ft_fs_1v8  "IO8_FT 166MHz HSLV fast speed @ 1.8V"
io8_166m_hslv_ft_fs_pu_1v8  "IO8_FT 166MHz HSLV fast speed @ 1.8V pullup"
io8_166m_hslv_ft_fs_pd_1v8  "IO8_FT 166MHz HSLV fast speed @ 1.8V pulldown"
io8_166m_hslv_ft_ms_1v8  "IO8_FT 166MHz HSLV med speed @ 1.8V"
io8_166m_hslv_ft_ms_pu_1v8  "IO8_FT 166MHz HSLV med speed @ 1.8V pullup"
io8_166m_hslv_ft_ms_pd_1v8  "IO8_FT 166MHz HSLV med speed @ 1.8V pulldown"
io8_166m_hslv_ft_ls_1v8  "IO8_FT 166MHz HSLV low speed @ 1.8V"
io8_166m_hslv_ft_ls_pu_1v8  "IO8_FT 166MHz HSLV low speed @ 1.8V pullup"
io8_166m_hslv_ft_ls_pd_1v8  "IO8_FT 166MHz HSLV low speed @ 1.8V pulldown"
io8_166m_hslv_ft_hs_2v5  "IO8_FT 166MHz HSLV high speed @ 2.5V"
io8_166m_hslv_ft_hs_pu_2v5  "IO8_FT 166MHz HSLV high speed @ 2.5V pullup"
io8_166m_hslv_ft_hs_pd_2v5  "IO8_FT 166MHz HSLV high speed @ 2.5V pulldown"
io8_166m_hslv_ft_fs_2v5  "IO8_FT 166MHz HSLV fast speed @ 2.5V"
io8_166m_hslv_ft_fs_pu_2v5  "IO8_FT 166MHz HSLV fast speed @ 2.5V pullup"
io8_166m_hslv_ft_fs_pd_2v5  "IO8_FT 166MHz HSLV fast speed @ 2.5V pulldown"
io8_166m_hslv_ft_ms_2v5  "IO8_FT 166MHz HSLV med speed @ 2.5V"
io8_166m_hslv_ft_ms_pu_2v5  "IO8_FT 166MHz HSLV med speed @ 2.5V pullup"
io8_166m_hslv_ft_ms_pd_2v5  "IO8_FT 166MHz HSLV med speed @ 2.5V pulldown"
io8_166m_hslv_ft_ls_2v5  "IO8_FT 166MHz HSLV low speed @ 2.5V"
io8_166m_hslv_ft_ls_pu_2v5  "IO8_FT 166MHz HSLV low speed @ 2.5V pullup"
io8_166m_hslv_ft_ls_pd_2v5  "IO8_FT 166MHz HSLV low speed @ 2.5V pulldown"
[Model Selector] io8_166m_hslv_i2c_ft
io8_166m_ft_hs_1v2  "IO8_FT 166MHz high speed @ 1.2V"
io8_166m_ft_hs_pu_1v2  "IO8_FT 166MHz high speed @ 1.2V pullup"
io8_166m_ft_hs_pd_1v2  "IO8_FT 166MHz high speed @ 1.2V pulldown"
io8_166m_ft_fs_1v2  "IO8_FT 166MHz fast speed @ 1.2V"
io8_166m_ft_fs_pu_1v2  "IO8_FT 166MHz fast speed @ 1.2V pullup"
io8_166m_ft_fs_pd_1v2  "IO8_FT 166MHz fast speed @ 1.2V pulldown"
io8_166m_ft_ms_1v2  "IO8_FT 166MHz med speed @ 1.2V"
io8_166m_ft_ms_pu_1v2  "IO8_FT 166MHz med speed @ 1.2V pullup"
io8_166m_ft_ms_pd_1v2  "IO8_FT 166MHz med speed @ 1.2V pulldown"
io8_166m_ft_ls_1v2  "IO8_FT 166MHz low speed @ 1.2V"
io8_166m_ft_ls_pu_1v2  "IO8_FT 166MHz low speed @ 1.2V pullup"
io8_166m_ft_ls_pd_1v2  "IO8_FT 166MHz low speed @ 1.2V pulldown"
io8_166m_ft_hs_1v8  "IO8_FT 166MHz high speed @ 1.8V"
io8_166m_ft_hs_pu_1v8  "IO8_FT 166MHz high speed @ 1.8V pullup"
io8_166m_ft_hs_pd_1v8  "IO8_FT 166MHz high speed @ 1.8V pulldown"
io8_166m_ft_fs_1v8  "IO8_FT 166MHz fast speed @ 1.8V"
io8_166m_ft_fs_pu_1v8  "IO8_FT 166MHz fast speed @ 1.8V pullup"
io8_166m_ft_fs_pd_1v8  "IO8_FT 166MHz fast speed @ 1.8V pulldown"
io8_166m_ft_ms_1v8  "IO8_FT 166MHz med speed @ 1.8V"
io8_166m_ft_ms_pu_1v8  "IO8_FT 166MHz med speed @ 1.8V pullup"
io8_166m_ft_ms_pd_1v8  "IO8_FT 166MHz med speed @ 1.8V pulldown"
io8_166m_ft_ls_1v8  "IO8_FT 166MHz low speed @ 1.8V"
io8_166m_ft_ls_pu_1v8  "IO8_FT 166MHz low speed @ 1.8V pullup"
io8_166m_ft_ls_pd_1v8  "IO8_FT 166MHz low speed @ 1.8V pulldown"
io8_166m_ft_hs_3v3  "IO8_FT 166MHz high speed @ 3.3V"
io8_166m_ft_hs_pu_3v3  "IO8_FT 166MHz high speed @ 3.3V pullup"
io8_166m_ft_hs_pd_3v3  "IO8_FT 166MHz high speed @ 3.3V pulldown"
io8_166m_ft_fs_3v3  "IO8_FT 166MHz fast speed @ 3.3V"
io8_166m_ft_fs_pu_3v3  "IO8_FT 166MHz fast speed @ 3.3V pullup"
io8_166m_ft_fs_pd_3v3  "IO8_FT 166MHz fast speed @ 3.3V pulldown"
io8_166m_ft_ms_3v3  "IO8_FT 166MHz med speed @ 3.3V"
io8_166m_ft_ms_pu_3v3  "IO8_FT 166MHz med speed @ 3.3V pullup"
io8_166m_ft_ms_pd_3v3  "IO8_FT 166MHz med speed @ 3.3V pulldown"
io8_166m_ft_ls_3v3  "IO8_FT 166MHz low speed @ 3.3V"
io8_166m_ft_ls_pu_3v3  "IO8_FT 166MHz low speed @ 3.3V pullup"
io8_166m_ft_ls_pd_3v3  "IO8_FT 166MHz low speed @ 3.3V pulldown"
io8_166m_hslv_ft_hs_1v2  "IO8_FT 166MHz HSLV high speed @ 1.2V"
io8_166m_hslv_ft_hs_pu_1v2  "IO8_FT 166MHz HSLV high speed @ 1.2V pullup"
io8_166m_hslv_ft_hs_pd_1v2  "IO8_FT 166MHz HSLV high speed @ 1.2V pulldown"
io8_166m_hslv_ft_fs_1v2  "IO8_FT 166MHz HSLV fast speed @ 1.2V"
io8_166m_hslv_ft_fs_pu_1v2  "IO8_FT 166MHz HSLV fast speed @ 1.2V pullup"
io8_166m_hslv_ft_fs_pd_1v2  "IO8_FT 166MHz HSLV fast speed @ 1.2V pulldown"
io8_166m_hslv_ft_ms_1v2  "IO8_FT 166MHz HSLV med speed @ 1.2V"
io8_166m_hslv_ft_ms_pu_1v2  "IO8_FT 166MHz HSLV med speed @ 1.2V pullup"
io8_166m_hslv_ft_ms_pd_1v2  "IO8_FT 166MHz HSLV med speed @ 1.2V pulldown"
io8_166m_hslv_ft_ls_1v2  "IO8_FT 166MHz HSLV low speed @ 1.2V"
io8_166m_hslv_ft_ls_pu_1v2  "IO8_FT 166MHz HSLV low speed @ 1.2V pullup"
io8_166m_hslv_ft_ls_pd_1v2  "IO8_FT 166MHz HSLV low speed @ 1.2V pulldown"
io8_166m_hslv_ft_hs_1v8  "IO8_FT 166MHz HSLV high speed @ 1.8V"
io8_166m_hslv_ft_hs_pu_1v8  "IO8_FT 166MHz HSLV high speed @ 1.8V pullup"
io8_166m_hslv_ft_hs_pd_1v8  "IO8_FT 166MHz HSLV high speed @ 1.8V pulldown"
io8_166m_hslv_ft_fs_1v8  "IO8_FT 166MHz HSLV fast speed @ 1.8V"
io8_166m_hslv_ft_fs_pu_1v8  "IO8_FT 166MHz HSLV fast speed @ 1.8V pullup"
io8_166m_hslv_ft_fs_pd_1v8  "IO8_FT 166MHz HSLV fast speed @ 1.8V pulldown"
io8_166m_hslv_ft_ms_1v8  "IO8_FT 166MHz HSLV med speed @ 1.8V"
io8_166m_hslv_ft_ms_pu_1v8  "IO8_FT 166MHz HSLV med speed @ 1.8V pullup"
io8_166m_hslv_ft_ms_pd_1v8  "IO8_FT 166MHz HSLV med speed @ 1.8V pulldown"
io8_166m_hslv_ft_ls_1v8  "IO8_FT 166MHz HSLV low speed @ 1.8V"
io8_166m_hslv_ft_ls_pu_1v8  "IO8_FT 166MHz HSLV low speed @ 1.8V pullup"
io8_166m_hslv_ft_ls_pd_1v8  "IO8_FT 166MHz HSLV low speed @ 1.8V pulldown"
io8_166m_hslv_ft_hs_2v5  "IO8_FT 166MHz HSLV high speed @ 2.5V"
io8_166m_hslv_ft_hs_pu_2v5  "IO8_FT 166MHz HSLV high speed @ 2.5V pullup"
io8_166m_hslv_ft_hs_pd_2v5  "IO8_FT 166MHz HSLV high speed @ 2.5V pulldown"
io8_166m_hslv_ft_fs_2v5  "IO8_FT 166MHz HSLV fast speed @ 2.5V"
io8_166m_hslv_ft_fs_pu_2v5  "IO8_FT 166MHz HSLV fast speed @ 2.5V pullup"
io8_166m_hslv_ft_fs_pd_2v5  "IO8_FT 166MHz HSLV fast speed @ 2.5V pulldown"
io8_166m_hslv_ft_ms_2v5  "IO8_FT 166MHz HSLV med speed @ 2.5V"
io8_166m_hslv_ft_ms_pu_2v5  "IO8_FT 166MHz HSLV med speed @ 2.5V pullup"
io8_166m_hslv_ft_ms_pd_2v5  "IO8_FT 166MHz HSLV med speed @ 2.5V pulldown"
io8_166m_hslv_ft_ls_2v5  "IO8_FT 166MHz HSLV low speed @ 2.5V"
io8_166m_hslv_ft_ls_pu_2v5  "IO8_FT 166MHz HSLV low speed @ 2.5V pullup"
io8_166m_hslv_ft_ls_pd_2v5  "IO8_FT 166MHz HSLV low speed @ 2.5V pulldown"
io8_166m_i2c_ft_1v2  "IO8_FT 166MHz I2C @ 1.2V"
io8_166m_i2c_ft_pu_1v2  "IO8_FT 166MHz I2C @ 1.2V pullup"
io8_166m_i2c_ft_pd_1v2  "IO8_FT 166MHz I2C @ 1.2V pulldown"
io8_166m_i2c_ft_1v8  "IO8_FT 166MHz I2C @ 1.8V"
io8_166m_i2c_ft_pu_1v8  "IO8_FT 166MHz I2C @ 1.8V pullup"
io8_166m_i2c_ft_pd_1v8  "IO8_FT 166MHz I2C @ 1,8V pulldown"
io8_166m_i2c_ft_3v3  "IO8_FT 166MHz I2C @ 3.3V"
io8_166m_i2c_ft_pu_3v3  "IO8_FT 166MHz I2C HSLV @ 3.3V pullup"
io8_166m_i2c_ft_pd_3v3  "IO8_FT 166MHz I2C @ 3.3V pulldown"
[Model Selector] io8_100m_ft_v33
io8_ft_v33_hs_1v2  "IO8_FT_V33 high speed @ 1.2V"
io8_ft_v33_hs_pu_1v2  "IO8_FT_V33 high speed @ 1.2V pullup"
io8_ft_v33_hs_pd_1v2  "IO8_FT_V33 high speed @ 1.2V pulldown"
io8_ft_v33_fs_1v2  "IO8_FT_V33 fast speed @ 1.2V"
io8_ft_v33_fs_pu_1v2  "IO8_FT_V33 fast speed @ 1.2V pullup"
io8_ft_v33_fs_pd_1v2  "IO8_FT_V33 fast speed @ 1.2V pulldown"
io8_ft_v33_ms_1v2  "IO8_FT_V33 med speed @ 1.2V"
io8_ft_v33_ms_pu_1v2  "IO8_FT_V33 med speed @ 1.2V pullup"
io8_ft_v33_ms_pd_1v2  "IO8_FT_V33 med speed @ 1.2V pulldown"
io8_ft_v33_ls_1v2  "IO8_FT_V33 low speed @ 1.2V"
io8_ft_v33_ls_pu_1v2  "IO8_FT_V33 low speed @ 1.2V pullup"
io8_ft_v33_ls_pd_1v2  "IO8_FT_V33 low speed @ 1.2V pulldown"
io8_ft_v33_hs_1v8  "IO8_FT_V33 high speed @ 1.8V"
io8_ft_v33_hs_pu_1v8  "IO8_FT_V33 high speed @ 1.8V pullup"
io8_ft_v33_hs_pd_1v8  "IO8_FT_V33 high speed @ 1.8V pulldown"
io8_ft_v33_fs_1v8  "IO8_FT_V33 fast speed @ 1.8V"
io8_ft_v33_fs_pu_1v8  "IO8_FT_V33 fast speed @ 1.8V pullup"
io8_ft_v33_fs_pd_1v8  "IO8_FT_V33 fast speed @ 1.8V pulldown"
io8_ft_v33_ms_1v8  "IO8_FT_V33 med speed @ 1.8V"
io8_ft_v33_ms_pu_1v8  "IO8_FT_V33 med speed @ 1.8V pullup"
io8_ft_v33_ms_pd_1v8  "IO8_FT_V33 med speed @ 1.8V pulldown"
io8_ft_v33_ls_1v8  "IO8_FT_V33 low speed @ 1.8V"
io8_ft_v33_ls_pu_1v8  "IO8_FT_V33 low speed @ 1.8V pullup"
io8_ft_v33_ls_pd_1v8  "IO8_FT_V33 low speed @ 1.8V pulldown"
io8_ft_v33_hs_3v3  "IO8_FT_V33 high speed @ 3.3V"
io8_ft_v33_hs_pu_3v3  "IO8_FT_V33 high speed @ 3.3V pullup"
io8_ft_v33_hs_pd_3v3  "IO8_FT_V33 high speed @ 3.3V pulldown"
io8_ft_v33_fs_3v3  "IO8_FT_V33 fast speed @ 3.3V"
io8_ft_v33_fs_pu_3v3  "IO8_FT_V33 fast speed @ 3.3V pullup"
io8_ft_v33_fs_pd_3v3  "IO8_FT_V33 fast speed @ 3.3V pulldown"
io8_ft_v33_ms_3v3  "IO8_FT_V33 med speed @ 3.3V"
io8_ft_v33_ms_pu_3v3  "IO8_FT_V33 med speed @ 3.3V pullup"
io8_ft_v33_ms_pd_3v3  "IO8_FT_V33 med speed @ 3.3V pulldown"
io8_ft_v33_ls_3v3  "IO8_FT_V33 low speed @ 3.3V"
io8_ft_v33_ls_pu_3v3  "IO8_FT_V33 low speed @ 3.3V pullup"
io8_ft_v33_ls_pd_3v3  "IO8_FT_V33 low speed @ 3.3V pulldown"
[Define Package Model]  455-qfpn-7x7-48-ldo-230504
[Manufacturer]  Unknown
[OEM]  Unknown
[Description]  None
[Number Of Pins]  46
[Pin Numbers]
| Pin Num   Terminal Name
7 | NRST
10 | PA0
31 | PA10
32 | PA11
33 | PA12
34 | PA13
37 | PA14
38 | PA15
11 | PA1
12 | PA2
13 | PA3
14 | PA4
15 | PA5
16 | PA6
17 | PA7
29 | PA8
30 | PA9
18 | PB0
21 | PB10
25 | PB12
26 | PB13
27 | PB14
28 | PB15
19 | PB1
20 | PB2
39 | PB3
40 | PB4
41 | PB5
42 | PB6
43 | PB7
45 | PB8
46 | PB9
2 | PC13
3 | PC14-OSC32_IN
4 | PC15-OSC32_OUT
5 | PH0-OSC_IN
6 | PH1-OSC_OUT
44 | PH3-BOOT0
22 | VCAP
1 | VBAT
24 | VDD
36 | VDD
48 | VDD
9 | VDDA
23 | VSS
8 | VSSA
|[Merged Pins]  23
|35  |  VSS
|47  |  VSS
[Model Data]
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[End Model Data]
[End Package Model]
| Models and submodels in the file (208): io8_100m_ft_hs_1v2 (I/O), io8_100m_ft_hs_pu_1v2 (I/O), io8_100m_ft_hs_pd_1v2 (I/O), io8_100m_ft_fs_1v2 (I/O), io8_100m_ft_fs_pu_1v2 (I/O), io8_100m_ft_fs_pd_1v2 (I/O), io8_100m_ft_ms_1v2 (I/O), io8_100m_ft_ms_pu_1v2 (I/O), io8_100m_ft_ms_pd_1v2 (I/O), io8_100m_ft_ls_1v2 (I/O), io8_100m_ft_ls_pu_1v2 (I/O), io8_100m_ft_ls_pd_1v2 (I/O), io8_100m_ft_hs_1v8 (I/O), io8_100m_ft_hs_pu_1v8 (I/O), io8_100m_ft_hs_pd_1v8 (I/O), io8_100m_ft_fs_1v8 (I/O), io8_100m_ft_fs_pu_1v8 (I/O), io8_100m_ft_fs_pd_1v8 (I/O), io8_100m_ft_ms_1v8 (I/O), io8_100m_ft_ms_pu_1v8 (I/O), io8_100m_ft_ms_pd_1v8 (I/O), io8_100m_ft_ls_1v8 (I/O), io8_100m_ft_ls_pu_1v8 (I/O), io8_100m_ft_ls_pd_1v8 (I/O), io8_100m_ft_hs_3v3 (I/O), io8_100m_ft_hs_pu_3v3 (I/O), io8_100m_ft_hs_pd_3v3 (I/O), io8_100m_ft_fs_3v3 (I/O), io8_100m_ft_fs_pu_3v3 (I/O), io8_100m_ft_fs_pd_3v3 (I/O), io8_100m_ft_ms_3v3 (I/O), io8_100m_ft_ms_pu_3v3 (I/O), io8_100m_ft_ms_pd_3v3 (I/O), io8_100m_ft_ls_3v3 (I/O), io8_100m_ft_ls_pu_3v3 (I/O), io8_100m_ft_ls_pd_3v3 (I/O), io8_100m_hslv_ft_hs_1v2 (I/O), io8_100m_hslv_ft_hs_pu_1v2 (I/O), io8_100m_hslv_ft_hs_pd_1v2 (I/O), io8_100m_hslv_ft_fs_1v2 (I/O), io8_100m_hslv_ft_fs_pu_1v2 (I/O), io8_100m_hslv_ft_fs_pd_1v2 (I/O), io8_100m_hslv_ft_ms_1v2 (I/O), io8_100m_hslv_ft_ms_pu_1v2 (I/O), io8_100m_hslv_ft_ms_pd_1v2 (I/O), io8_100m_hslv_ft_ls_1v2 (I/O), io8_100m_hslv_ft_ls_pu_1v2 (I/O), io8_100m_hslv_ft_ls_pd_1v2 (I/O), io8_100m_hslv_ft_hs_1v8 (I/O), io8_100m_hslv_ft_hs_pu_1v8 (I/O), io8_100m_hslv_ft_hs_pd_1v8 (I/O), io8_100m_hslv_ft_fs_1v8 (I/O), io8_100m_hslv_ft_fs_pu_1v8 (I/O), io8_100m_hslv_ft_fs_pd_1v8 (I/O), io8_100m_hslv_ft_ms_1v8 (I/O), io8_100m_hslv_ft_ms_pu_1v8 (I/O), io8_100m_hslv_ft_ms_pd_1v8 (I/O), io8_100m_hslv_ft_ls_1v8 (I/O), io8_100m_hslv_ft_ls_pu_1v8 (I/O), io8_100m_hslv_ft_ls_pd_1v8 (I/O), io8_100m_hslv_ft_hs_2v5 (I/O), io8_100m_hslv_ft_hs_pu_2v5 (I/O), io8_100m_hslv_ft_hs_pd_2v5 (I/O), io8_100m_hslv_ft_fs_2v5 (I/O), io8_100m_hslv_ft_fs_pu_2v5 (I/O), io8_100m_hslv_ft_fs_pd_2v5 (I/O), io8_100m_hslv_ft_ms_2v5 (I/O), io8_100m_hslv_ft_ms_pu_2v5 (I/O), io8_100m_hslv_ft_ms_pd_2v5 (I/O), io8_100m_hslv_ft_ls_2v5 (I/O), io8_100m_hslv_ft_ls_pu_2v5 (I/O), io8_100m_hslv_ft_ls_pd_2v5 (I/O), io8_166m_ft_hs_1v2 (I/O), io8_166m_ft_hs_pu_1v2 (I/O), io8_166m_ft_hs_pd_1v2 (I/O), io8_166m_ft_fs_1v2 (I/O), io8_166m_ft_fs_pu_1v2 (I/O), io8_166m_ft_fs_pd_1v2 (I/O), io8_166m_ft_ms_1v2 (I/O), io8_166m_ft_ms_pu_1v2 (I/O)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
